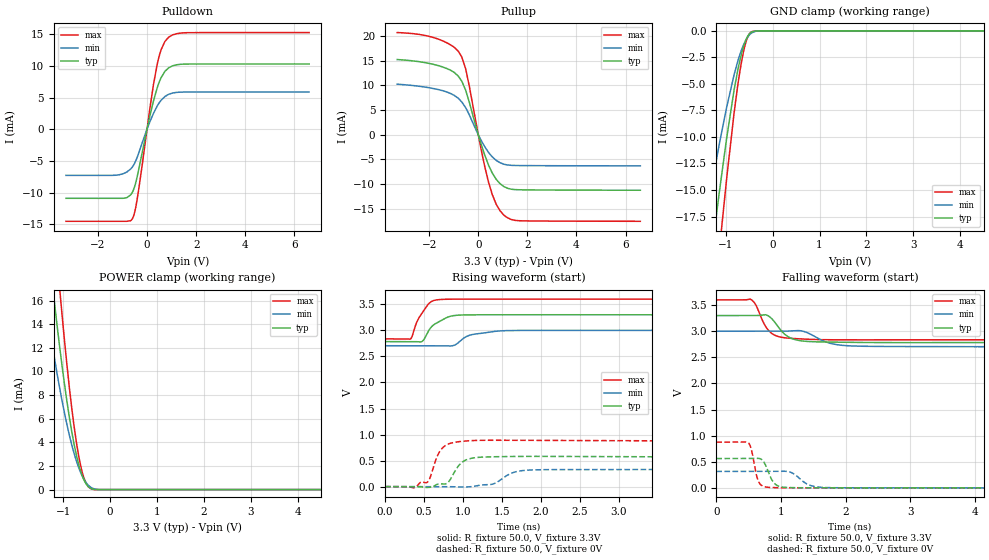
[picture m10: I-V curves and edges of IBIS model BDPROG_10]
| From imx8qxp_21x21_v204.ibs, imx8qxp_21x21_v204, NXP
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[Model]   BDPROG_10
Model_type I/O
Polarity   Non-Inverting
Enable   Active-Low
| CAP_THRESHOLD on pad IO is "CMOS" :
| Rising=10.0% of vdde3v3   Falling=90.0% of vdde3v3
| C_comp min and max val. don't necessarily correlate with the min and max pvt
| but are the smallest and greatest pad capacitance found.
| var   typ   min   max
C_comp   1.85655pF  1.66230pF  1.93185pF
Vinl = 800.0mV
Vinh = 2.0V
Vmeas = 1.65V   | Reference voltage for timing measurements
Cref  = 50.0pF   | Timing specification test load capacitance value
Rref  = 1.0MOhm   | Timing specification test load resistance value
Vref  = 3.3V   | Timing specification test load voltage
[Model Spec]
| TIME_THRESHOLD on pin ZI is "CORE" :
| Rising=50.0% of vdd   Falling=50.0% of vdd
Vinl 800.00000mV 800.00000mV 800.00000mV
Vinh 2.00000V 2.00000V 2.00000V
Vmeas 1.65000V 1.50000V 1.80000V
Vref 3.30000V 3.00000V 3.60000V
| variable   typ   min   max
[Temperature Range] 25.0 125.0 -40.0
| variable   typ   min   max
[Voltage Range] 3.3V 3.0V 3.6V
| variable   typ   min   max
[POWER Clamp Reference] 3.3V 3.0V 3.6V
| variable   typ   min   max
[GND Clamp Reference] 0V 0V 0V
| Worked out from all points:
|   slope of the pulldown table from 0 to 0.495 V, typ, clamps not added: 66.7 ohm
|   slope of the pullup table from 0 to 0.495 V, typ, clamps not added: 71 ohm
|   GND clamp passes 1 mA (typ) near -0.58 V on its own axis
|   POWER clamp passes 1 mA (typ) near -0.58 V on its own axis
|   rising waveform, R_fixture 50.0, V_fixture 3.3V: 20-80 % time 209ps typ, 280ps min, 159ps max; typ from 2.79 V to 3.3 V
|   falling waveform, R_fixture 50.0, V_fixture 3.3V: 20-80 % time 231ps typ, 315ps min, 194ps max; typ from 3.3 V to 2.79 V
|   rising waveform, R_fixture 50.0, V_fixture 0V: 20-80 % time 147ps typ, 204ps min, 135ps max; typ from 0 V to 0.561 V
|   falling waveform, R_fixture 50.0, V_fixture 0V: 20-80 % time 124ps typ, 202ps min, 87.4ps max; typ from 0.561 V to 0 V
[POWER Clamp]
-3.3V     110.4mA    79.71mA    140.4mA
-1.39V    23.37mA    16.28mA    32.13mA
-1.23V    17.37mA    12.17mA    24.18mA
-1.18V    15.59mA    10.96mA    21.8mA
-1.08V    12.22mA    8.693mA    17.21mA
-1.02V    10.33mA    7.426mA    14.59mA
-870mV    6.147mA    4.623mA    8.679mA
-710mV    2.758mA    2.312mA    3.771mA
-610mV    1.329mA    1.277mA    1.706mA
-560mV    827.2uA    884.9uA    1.001mA
-400mV    73.97uA    165.7uA    50.71uA
6.6V      0A         0A         0A
[GND Clamp]
-3.3V     -81.81mA   -63.72mA   -95.03mA
-1.44V    -25.76mA   -18.09mA   -33.96mA
-1.29V    -20.51mA   -14.35mA   -27.46mA
-1.13V    -15.01mA   -10.53mA   -20.42mA
-980mV    -10.12mA   -7.21mA    -13.93mA
-820mV    -5.543mA   -4.118mA   -7.691mA
-690mV    -2.659mA   -2.142mA   -3.617mA
-570mV    -870.5uA   -872.8uA   -1.079mA
-510mV    -367.8uA   -465.5uA   -395.3uA
-450mV    -106.6uA   -203.3uA   -84.64uA
-200mV    -18.65nA   -455.7nA   -5.392nA
6.6V      19.28nA    1.199uA    15.29nA
| variable   typ   min   max
[Pullup Reference] 3.3V 3.0V 3.6V
| variable   typ   min   max
[Pulldown Reference] 0V 0V 0V
[Pullup]
-3.3V     15.22mA    10.23mA    20.69mA
-2.39V    14.78mA    9.795mA    20.3mA
-1.6V     13.95mA    9.107mA    19.32mA
-980mV    12.62mA    7.966mA    17.71mA
-670mV    10.82mA    6.622mA    15.73mA
-510mV    8.966mA    5.447mA    13.28mA
110mV     -1.829mA   -1.09mA    -2.829mA
420mV     -6.185mA   -3.612mA   -9.654mA
730mV     -9.048mA   -5.209mA   -14.09mA
1.04V     -10.51mA   -5.982mA   -16.3mA
1.65V     -11.16mA   -6.254mA   -17.44mA
6.6V      -11.26mA   -6.316mA   -17.56mA
[Pulldown]
-3.3V     -10.9mA    -7.28mA    -14.53mA
-1.13V    -10.9mA    -7.184mA   -14.53mA
-820mV    -10.79mA   -6.749mA   -14.53mA
-590mV    -9.898mA   -5.919mA   -14.07mA
-490mV    -8.863mA   -5.246mA   -12.89mA
-380mV    -7.117mA   -4.218mA   -10.53mA
110mV     1.969mA    1.113mA    3.106mA
410mV     6.479mA    3.628mA    10.15mA
580mV     8.187mA    4.602mA    12.61mA
880mV     9.695mA    5.514mA    14.53mA
1.65V     10.29mA    5.871mA    15.24mA
6.6V      10.3mA     5.882mA    15.26mA
[Ramp]
dV/dt_r 336.5291mV/146.96484ps 188.63825mV/204.17371ps 525.27059mV/134.87594ps
dV/dt_f 308.92166mV/231.42321ps 176.32984mV/314.53756ps 457.66455mV/194.24911ps
R_load = 50.0
| Removed startup time: 0s 0s 0s  .
| Removed end time: 5.0ns.
[Rising Waveform]
R_fixture   = 50.0
V_fixture   = 3.3V
V_fixture_min = 3.0V
V_fixture_max = 3.6V
0s        2.785V     2.706V     2.837V
327ps     2.785V     2.706V     2.838V
410ps     2.783V     2.706V     3.169V
471ps     2.785V     2.706V     3.324V
535ps     2.929V     2.706V     3.466V
684ps     3.16V      2.706V     3.591V
893ps     3.287V     2.718V     3.601V
1.09ns    3.299V     2.91V      3.601V
1.507ns   3.301V     2.993V     3.601V
5ns       3.3V       3.001V     3.6V
| Removed startup time: 0s 0s 0s  .
| Removed end time: 20.0ns.
[Falling Waveform]
R_fixture   = 50.0
V_fixture   = 3.3V
V_fixture_min = 3.0V
V_fixture_max = 3.6V
0s        3.3V       3V         3.6V
528ps     3.3V       3V         3.613V
612ps     3.3V       3V         3.501V
764ps     3.315V     3V         3.087V
876ps     3.216V     3V         2.943V
1.132ns   2.88V      3.004V     2.866V
1.516ns   2.798V     2.903V     2.842V
1.864ns   2.79V      2.743V     2.836V
2.464ns   2.783V     2.709V     2.835V
20ns      2.785V     2.706V     2.837V
| Removed startup time: 0s 0s 0s  .
| Removed end time: 20.0ns.
[Rising Waveform]
R_fixture   = 50.0
V_fixture   = 0V
V_fixture_min = 0V
V_fixture_max = 0V
0s        38.9nV     696nV      70.27nV
536ps     -16.61mV   -3.01uV    78.38mV
676ps     47.48mV    23.98uV    604.7mV
752ps     49.19mV    376.8uV    764mV
980ps     457.9mV    -10.58mV   868.6mV
1.156ns   555.5mV    9.253mV    886.7mV
1.392ns   573.3mV    53.45mV    890.7mV
1.692ns   579.7mV    290.2mV    889.4mV
2.036ns   580.7mV    325.5mV    886.9mV
20ns      560.9mV    314.4mV    875.5mV
| Removed startup time: 0s 0s 0s  .
| Removed end time: 4.999ns.
[Falling Waveform]
R_fixture   = 50.0
V_fixture   = 0V
V_fixture_min = 0V
V_fixture_max = 0V
0s        560.9mV    314.3mV    875.5mV
495ps     560.9mV    314.4mV    864.4mV
544ps     561.4mV    314.4mV    723.5mV
644ps     565.3mV    314.4mV    146.7mV
762ps     433.2mV    314.5mV    16.13mV
892ps     93.15mV    314.8mV    4.025mV
1.068ns   8.684mV    316.8mV    933.4uV
1.426ns   654.7uV    59.14mV    -485.3uV
1.624ns   -15.84uV   9.4mV      -533.7uV
4.999ns   -151.1uV   -446.3uV   -25.03uV
